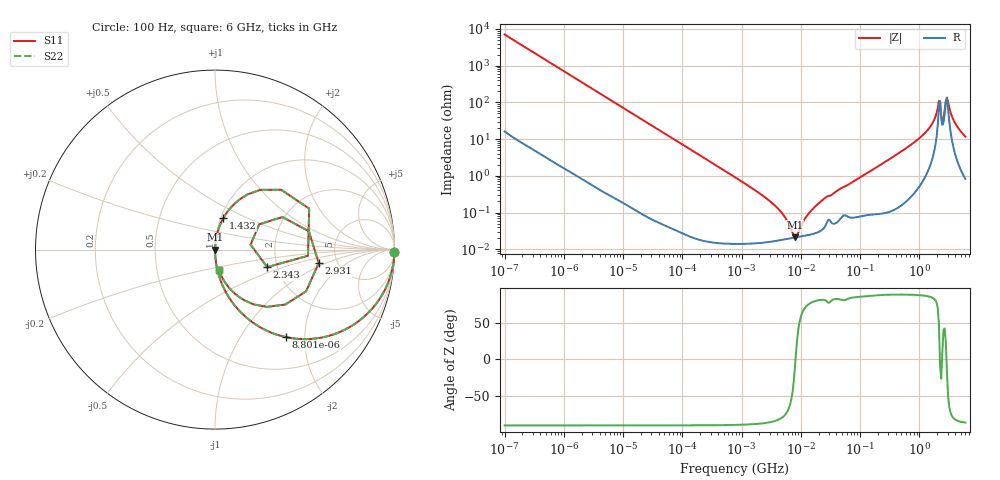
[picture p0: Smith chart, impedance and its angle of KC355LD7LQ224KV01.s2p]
!Murata Part Number: KC355LD7LQ224KV01
!These Parameters are Measured in Series Mode Connection
!Data Generated on Jun 19, 2026
!  o--ll--o
!Port1  Port2
!  o------o
!Operation Temp=25[degC], DC Bias Voltage=0[V]
!Freq. Start=100[Hz] Stop=6[GHz] 401[Steps]
# Hz S RI R 50
!Freq.(Hz) S11(Real) S11(Imag) S21(Real) S21(Imag) S12(Real) S12(Imag) S22(Real) S22(Imag)
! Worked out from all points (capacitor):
!   401 points, 100 Hz to 6 GHz, reference 50 ohm
!   read as one part in series: C = 225 nF near 109 Hz
!   lowest |Z| = 21.1 mohm at 7.948 MHz (marker M1)
!   series resonance near 8.14 MHz, so ESL is about 1.7 nH
!   S11 on the Smith chart (normalised r, x): 100 Hz: open; 8.801 kHz: 1.00, -1.62; 1.432 GHz: 1.03, +0.38; 2.343 GHz: 1.77, -0.38; 2.931 GHz: 3.59, -0.82; 6 GHz: 1.02, -0.23
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100  0.9998 -0.0141  0.000232 0.0141  0.000232 0.0141  0.9998 -0.0141
2008  0.9256 -0.2613  0.0744 0.2613  0.0744 0.2613  0.9256 -0.2613
3931  0.7656 -0.4224  0.2344 0.4224  0.2344 0.4224  0.7656 -0.4224
8801  0.3961 -0.4878  0.6039 0.4878  0.6039 0.4878  0.3961 -0.4878
18016  0.1361 -0.3416  0.8639 0.3416  0.8639 0.3416  0.1361 -0.3416
40335  0.0309 -0.1715  0.9691 0.1715  0.9691 0.1715  0.0309 -0.1715
774597  0.000223 -0.00915  0.9998 0.00915  0.9998 0.00915  0.000223 -0.00915
3882480  0.000171 -0.0014  0.9998 0.0014  0.9998 0.0014  0.000171 -0.0014
5554849  0.000188 -0.000672  0.9998 0.000672  0.9998 0.000672  0.000188 -0.000672
7947587  0.000207 -4.04e-05  0.9998 4.04e-05  0.9998 4.04e-05  0.000207 -4.04e-05
1.555665e7  0.000258 0.00118  0.9997 -0.00118  0.9997 -0.00118  0.000258 0.00118
2.662322e7  0.000474 0.00257  0.9995 -0.00257  0.9995 -0.00257  0.000474 0.00257
3.124326e8  0.00184 0.0282  0.9982 -0.0282  0.9982 -0.0282  0.00184 0.0282
1.431855e9  0.0473 0.177  0.9527 -0.177  0.9527 -0.177  0.0473 0.177
1.791126e9  0.1347 0.2778  0.8653 -0.2778  0.8653 -0.2778  0.1347 0.2778
2.048624e9  0.3688 0.3334  0.6312 -0.3334  0.6312 -0.3334  0.3688 0.3334
2.34314e9  0.2907 -0.0976  0.7093 0.0976  0.7093 0.0976  0.2907 -0.0976
2.679998e9  0.3757 0.1813  0.6243 -0.1813  0.6243 -0.1813  0.3757 0.1813
2.931063e9  0.5779 -0.075  0.4221 0.075  0.4221 0.075  0.5779 -0.075
3.505958e9  0.2158 -0.3054  0.7842 0.3054  0.7842 0.3054  0.2158 -0.3054
4.193612e9  0.0807 -0.2153  0.9193 0.2153  0.9193 0.2153  0.0807 -0.2153
6e9  0.0212 -0.1129  0.9788 0.1129  0.9788 0.1129  0.0212 -0.1129
